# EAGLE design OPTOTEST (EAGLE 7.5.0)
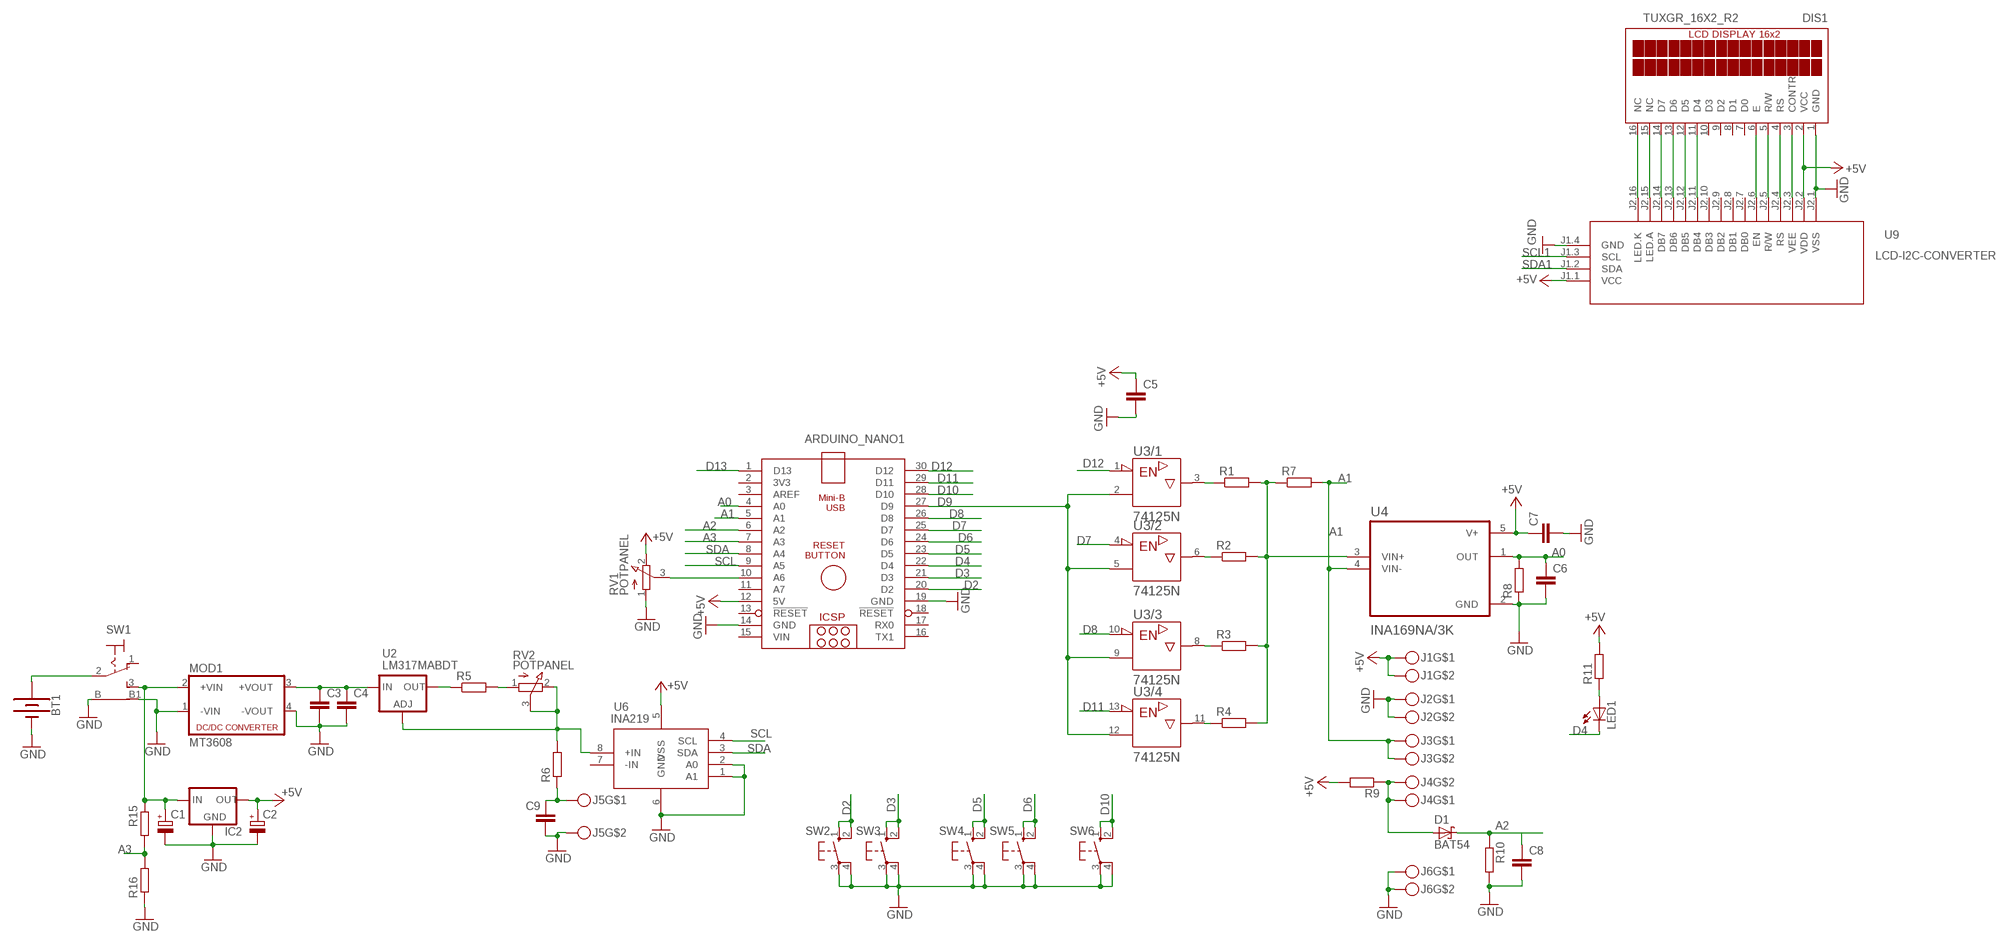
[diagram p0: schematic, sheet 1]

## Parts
ARDUINO_NANO1  ARDUINO_NANO  [ARDUINO_NANO]
BT1  BATTERY-9V  [BATTCON_9V]
C1  CPOL-EUSMCC  [SMC_C]
C2  CPOL-EUSMCC  [SMC_C]
C3  C-EUC1206  [C1206]
C4  C-EUC1206  [C1206]
C5  C-EUC1206  [C1206]
C6  C-EUC1206  [C1206]
C7  C-EUC1206  [C1206]
C8  C-EUC1206  [C1206]
C9  C-EUC1206  [C1206]
D1  BAT54  [SOT23]
DIS1  TUXGR_16X2_R2  [TUXGR_16X2_R2]
IC2  78XXL  [78XXL]
J1  MKDSN1,5-2-5,08  [MKDSN1,5-2-5,08]
J2  MKDSN1,5-2-5,08  [MKDSN1,5-2-5,08]
J3  MKDSN1,5-2-5,08  [MKDSN1,5-2-5,08]
J4  MKDSN1,5-2-5,08  [MKDSN1,5-2-5,08]
J5  MKDSN1,5-2-5,08  [MKDSN1,5-2-5,08]
J6  MKDSN1,5-2-5,08  [MKDSN1,5-2-5,08]
LED1  LED5MM  [LED5MM]
MOD1  MT3608  [MT3608]
R1  R-EU_R1206  [R1206]
R2  R-EU_R1206  [R1206]
R3  R-EU_R1206  [R1206]
R4  R-EU_R1206  [R1206]
R5  R-EU_R2512  [R2512]
R6  R-EU_R2512  [R2512]
R7  R-EU_R1206  [R1206]
R8  R-EU_R1206  [R1206]
R9  R-EU_R1206  [R1206]
R10  R-EU_R1206  [R1206]
R11  R-EU_R1206  [R1206]
R15  R-EU_R1206  [R1206]
R16  R-EU_R1206  [R1206]
RV1  POTPANEL  [POTPANELP231]
RV2  POTPANEL  [POTPANELP231]
SW1  9070-1W  [9070-1W]
SW2  40-XX  [B3F-40XX]
SW3  40-XX  [B3F-40XX]
SW4  40-XX  [B3F-40XX]
SW5  40-XX  [B3F-40XX]
SW6  40-XX  [B3F-40XX]
U2  LM317MABDT  [DPACK]
U3  74125N  [DIL14]
U4  INA169NA/3K  [SOT95P280X145-5N]
U6  INA219  [SO08]
U9  LCD-I2C-CONVERTER  [LCD-I2C-CONVERTER]

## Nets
+5V: ARDUINO_NANO1.12(5V) C2.+ C5.1 C7.1 DIS1.2(VCC) IC2.OUT J1.1 J1.2 R9.2 R11.2 RV1.2(E) U4.5(V+) U6.5(VSS) U9.J1.1(VCC) U9.J2.2(VDD)
A0: ARDUINO_NANO1.4(A0) C6.1 R8.2 U4.1(OUT)
A1: ARDUINO_NANO1.5(A1) J3.1 J3.2 R7.2 U4.4(VIN-)
A2: ARDUINO_NANO1.6(A2) C8.1 D1.3(C) R10.1
A3: ARDUINO_NANO1.7(A3) R15.1 R16.2
D2: ARDUINO_NANO1.20(D2) SW2.1(S) SW2.2(S1)
D3: ARDUINO_NANO1.21(D3) SW3.1(S) SW3.2(S1)
D4: ARDUINO_NANO1.22(D4) LED1.K(C)
D5: ARDUINO_NANO1.23(D5) SW4.1(S) SW4.2(S1)
D6: ARDUINO_NANO1.24(D6) SW5.1(S) SW5.2(S1)
D7: ARDUINO_NANO1.25(D7) U3.4(/2:!G)
D8: ARDUINO_NANO1.26(D8) U3.10(/3:!G)
D9: ARDUINO_NANO1.27(D9) U3.2(/1:A) U3.5(/2:A) U3.9(/3:A) U3.12(/4:A)
D10: ARDUINO_NANO1.28(D10) SW6.1(S) SW6.2(S1)
D11: ARDUINO_NANO1.29(D11) U3.13(/4:!G)
D12: ARDUINO_NANO1.30(D12) U3.1(/1:!G)
D13: ARDUINO_NANO1.1(D13)
GND: ARDUINO_NANO1.14(GND) ARDUINO_NANO1.19(GND) BT1.- C1.- C2.- C3.2 C4.2 C5.2 C6.2 C7.2 C8.2 C9.2 DIS1.1(GND) IC2.GND J2.1 J2.2 J5.2 J6.1 J6.2 MOD1.1(-VIN) MOD1.4(-VOUT) R8.1 R10.2 R16.1 RV1.1(A) SW1.B SW1.B1 SW2.3(P) SW2.4(P1) SW3.3(P) SW3.4(P1) SW4.3(P) SW4.4(P1) SW5.3(P) SW5.4(P1) SW6.3(P) SW6.4(P1) U4.2(GND) U6.1(A1) U6.2(A0) U6.6(GND) U9.J1.4(GND) U9.J2.1(VSS)
N$1: ARDUINO_NANO1.10(A6) RV1.3(S)
N$2: D1.1(A) J4.1 J4.2 R9.1
N$3: R1.1 U3.3(/1:Y)
N$4: R2.1 U3.6(/2:Y)
N$5: R3.1 U3.8(/3:Y)
N$6: R4.1 U3.11(/4:Y)
N$7: R1.2 R2.2 R3.2 R4.2 R7.1 U4.3(VIN+)
N$8: LED1.A R11.1
N$14: C3.1 C4.1 MOD1.3(+VOUT) U2.3(IN)
N$15: R5.1 U2.4(OUT)
N$16: R5.2 RV2.1(A)
N$17: R6.2 RV2.2(E) RV2.3(S) U2.1(ADJ) U6.8(+IN)
N$18: C1.+ IC2.IN MOD1.2(+VIN) R15.2 SW1.3(S)
N$19: C9.1 J5.1 R6.1
N$21: BT1.+ SW1.2(P)
N$31: DIS1.3(CONTR) U9.J2.3(VEE)
N$32: DIS1.4(RS) U9.J2.4(RS)
N$33: DIS1.5(R/W) U9.J2.5(R/W)
N$34: DIS1.6(E) U9.J2.6(EN)
N$35: DIS1.14(D7) U9.J2.14(DB7)
N$36: DIS1.13(D6) U9.J2.13(DB6)
N$37: DIS1.12(D5) U9.J2.12(DB5)
N$38: DIS1.11(D4) U9.J2.11(DB4)
N$39: DIS1.16(NC) U9.J2.16(LED.K)
N$40: DIS1.15(NC) U9.J2.15(LED.A)
SCL: ARDUINO_NANO1.9(A5) U6.4(SCL)
SCL1: U9.J1.3(SCL)
SDA: ARDUINO_NANO1.8(A4) U6.3(SDA)
SDA1: U9.J1.2(SDA)
Unconnected: ARDUINO_NANO1.2(3V3) ARDUINO_NANO1.3(AREF) ARDUINO_NANO1.11(A7) ARDUINO_NANO1.13(!RESET) ARDUINO_NANO1.16(TX1) ARDUINO_NANO1.17(RX0) ARDUINO_NANO1.18(!RESET) DIS1.7(D0) DIS1.8(D1) DIS1.9(D2) DIS1.10(D3) SW1.1(O) U6.7(-IN) U9.J2.7(DB0) U9.J2.8(DB1) U9.J2.9(DB2) U9.J2.10(DB3)

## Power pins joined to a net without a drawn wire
+UB: U3.14(/+UB:+UB)
-UB: U3.7(/-UB:-UB)
VIN: ARDUINO_NANO1.15(VIN)

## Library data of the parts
ARDUINO_NANO1 = ArduinoNanoV30:ARDUINO_NANO: Arduino Nano V3.0 Overview: The Arduino Nano is a small, complete, and breadboard-friendly board based on the ATmega328 (Arduino Nano 3.x) or ATmega168 (Arduino Nano 2.x). It has more or less the same functionality of the Arduino Duemilanove, but in a different package. It lacks only a DC power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
BT1 = SparkFun-Batteries:BATTERY: Battery - Single Cell; PROD_ID: BATT-10855
C1 C2 = rcl:CPOL-EU: POLARIZED CAPACITOR, European symbol
C3-C9 = rcl:C-EU: CAPACITOR, European symbol
D1 = diode:BAT54: Schottky Diodes
DIS1 = display-lcd:TUXGR_16X2_R2: Tuxgraphics LCD display 16x2 characters reflective, without background light Source: tuxgr_12x2_r2.pdf; OC_FARNELL: unknown; OC_NEWARK: unknown
IC2 = v-reg:78XXL: VOLTAGE REGULATOR
J1-J6 = con-phoenix-508:MKDSN1,5-2-5,08
LED1 = led:LED: LED
MOD1 = dc-dc-converter:MT3608: DC DC Up Converter
R1-R11 R15 R16 = rcl:R-EU_: RESISTOR, European symbol
RV1 RV2 = pot:POTPANEL
SW1 = switch:9070-1W: TOGGLE SWITCH Marquardt
SW2-SW6 = switch-omron:40-XX: OMRON SWITCH; MF: OMRON COMPONENTS USA; MPN: B3F-4000; OC_FARNELL: 176434; OC_NEWARK: 36K3105
U2 = v-reg:LM317?*: 500 mA Adjustable Output Positive Voltage Regulator Source: http://www.onsemi.co.jp .. LM317M-D.PDF
U3 = 74ttl-din:74*125: Quad bus BUFFER, 3-state
U4 = INA169NA_3K:INA169NA/3K: Check availability; AVAILABILITY: In Stock; CHECK_PRICES: https://www.snapeda.com/parts/INA169NA/3K/Texas+Instruments/view-part/?ref=eda; DESCRIPTION: 2.7 to 60V, 440kHz Variable gain current sense amplifier; MF: Texas Instruments; MP: INA169NA/3K; PACKAGE: SOT-23-5 Texas Instruments; PRICE: None; PURCHASE-URL: https://pricing.snapeda.com/search?q=INA169NA/3K&ref=eda; SNAPEDA_LINK: https://www.snapeda.com/parts/INA169NA/3K/Texas+Instruments/view-part/?ref=snap
U6 = burr-brown:INA219: Bidirectional Current/Power Monitor With I2C Interface
U9 = diy-modules:LCD-I2C-CONVERTER: I2C Bus to 4-Bit Parallel LCD Interface with LED backlight driver

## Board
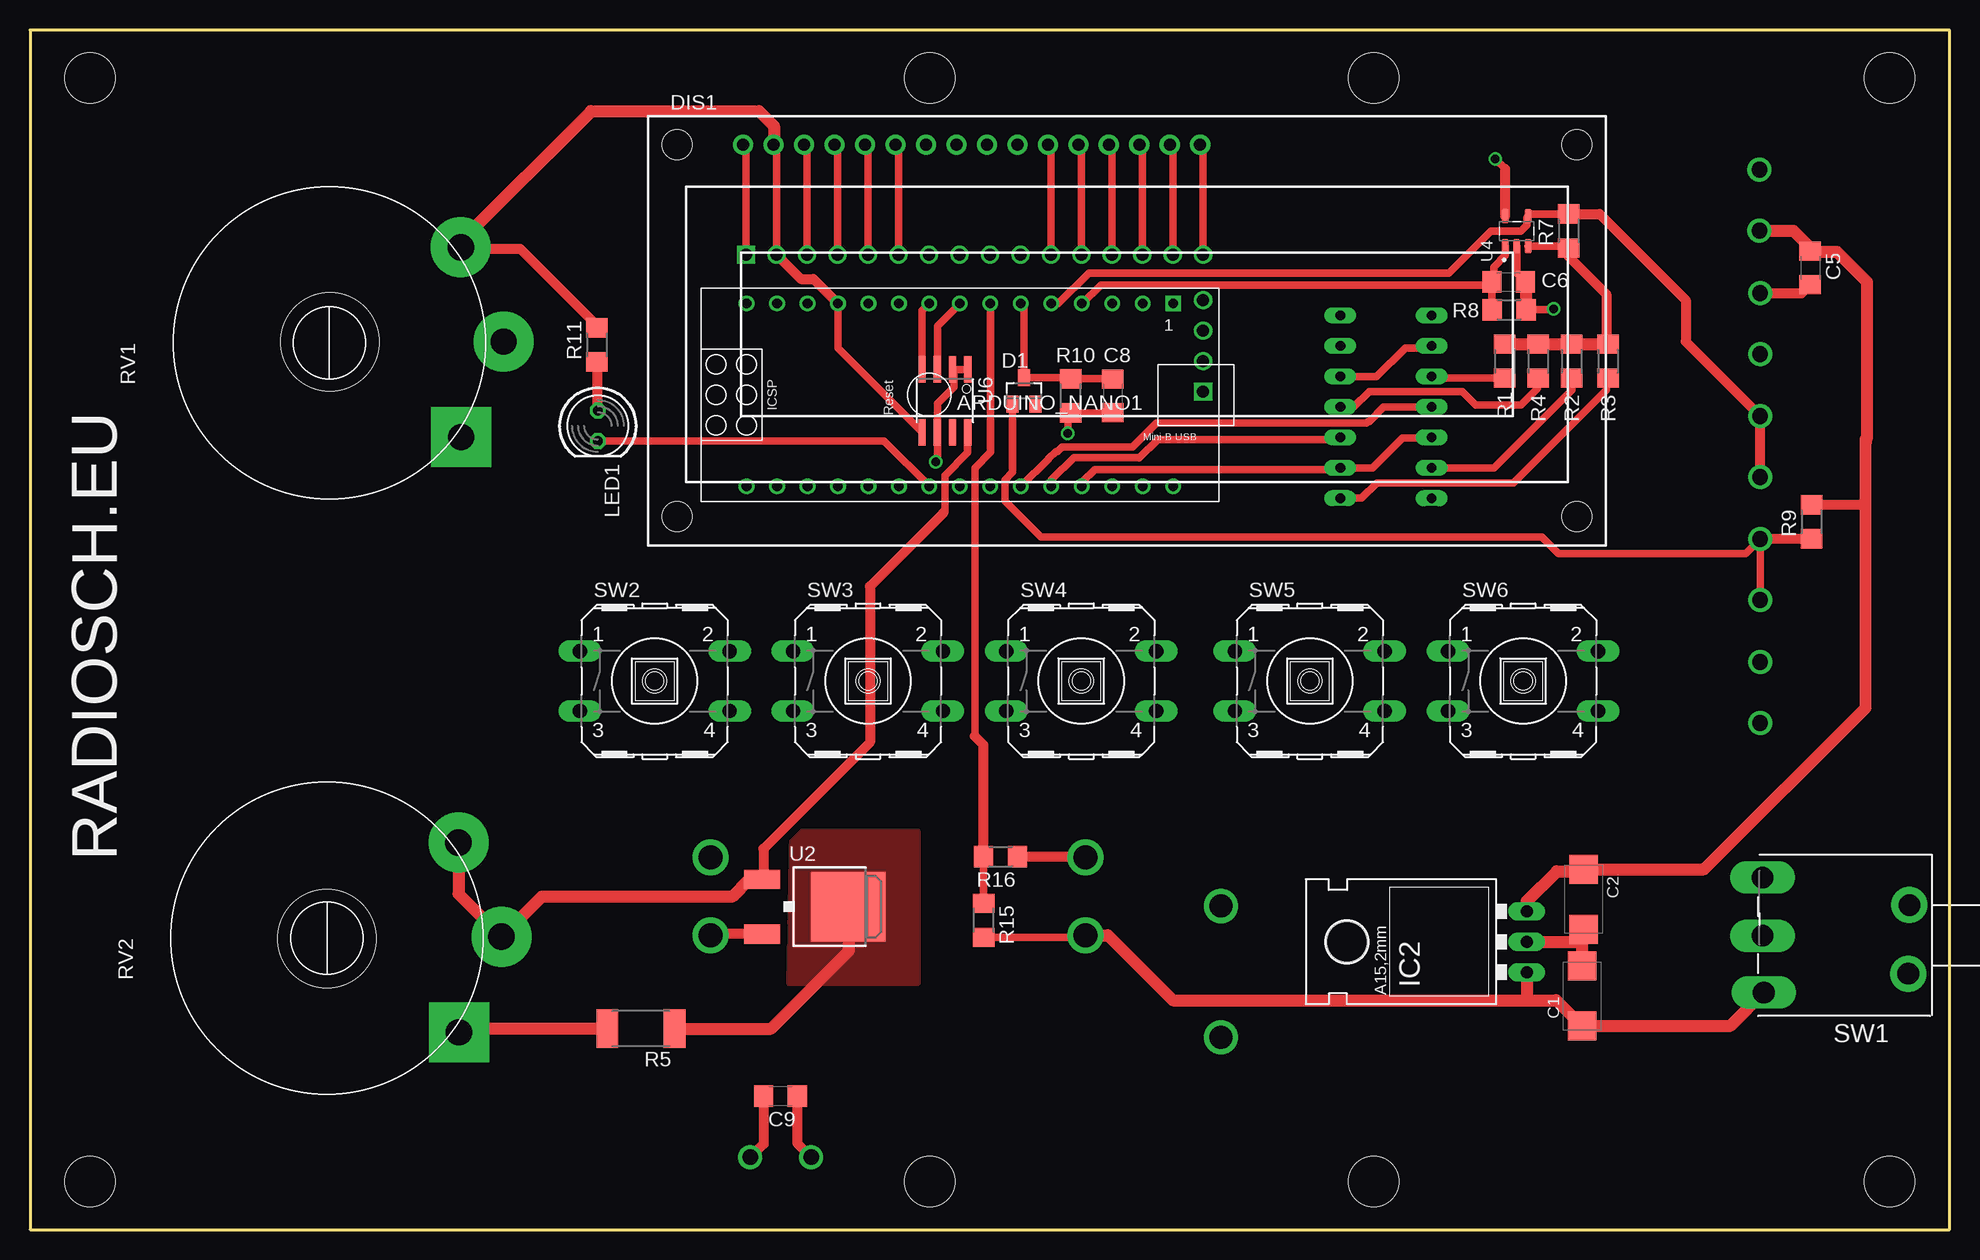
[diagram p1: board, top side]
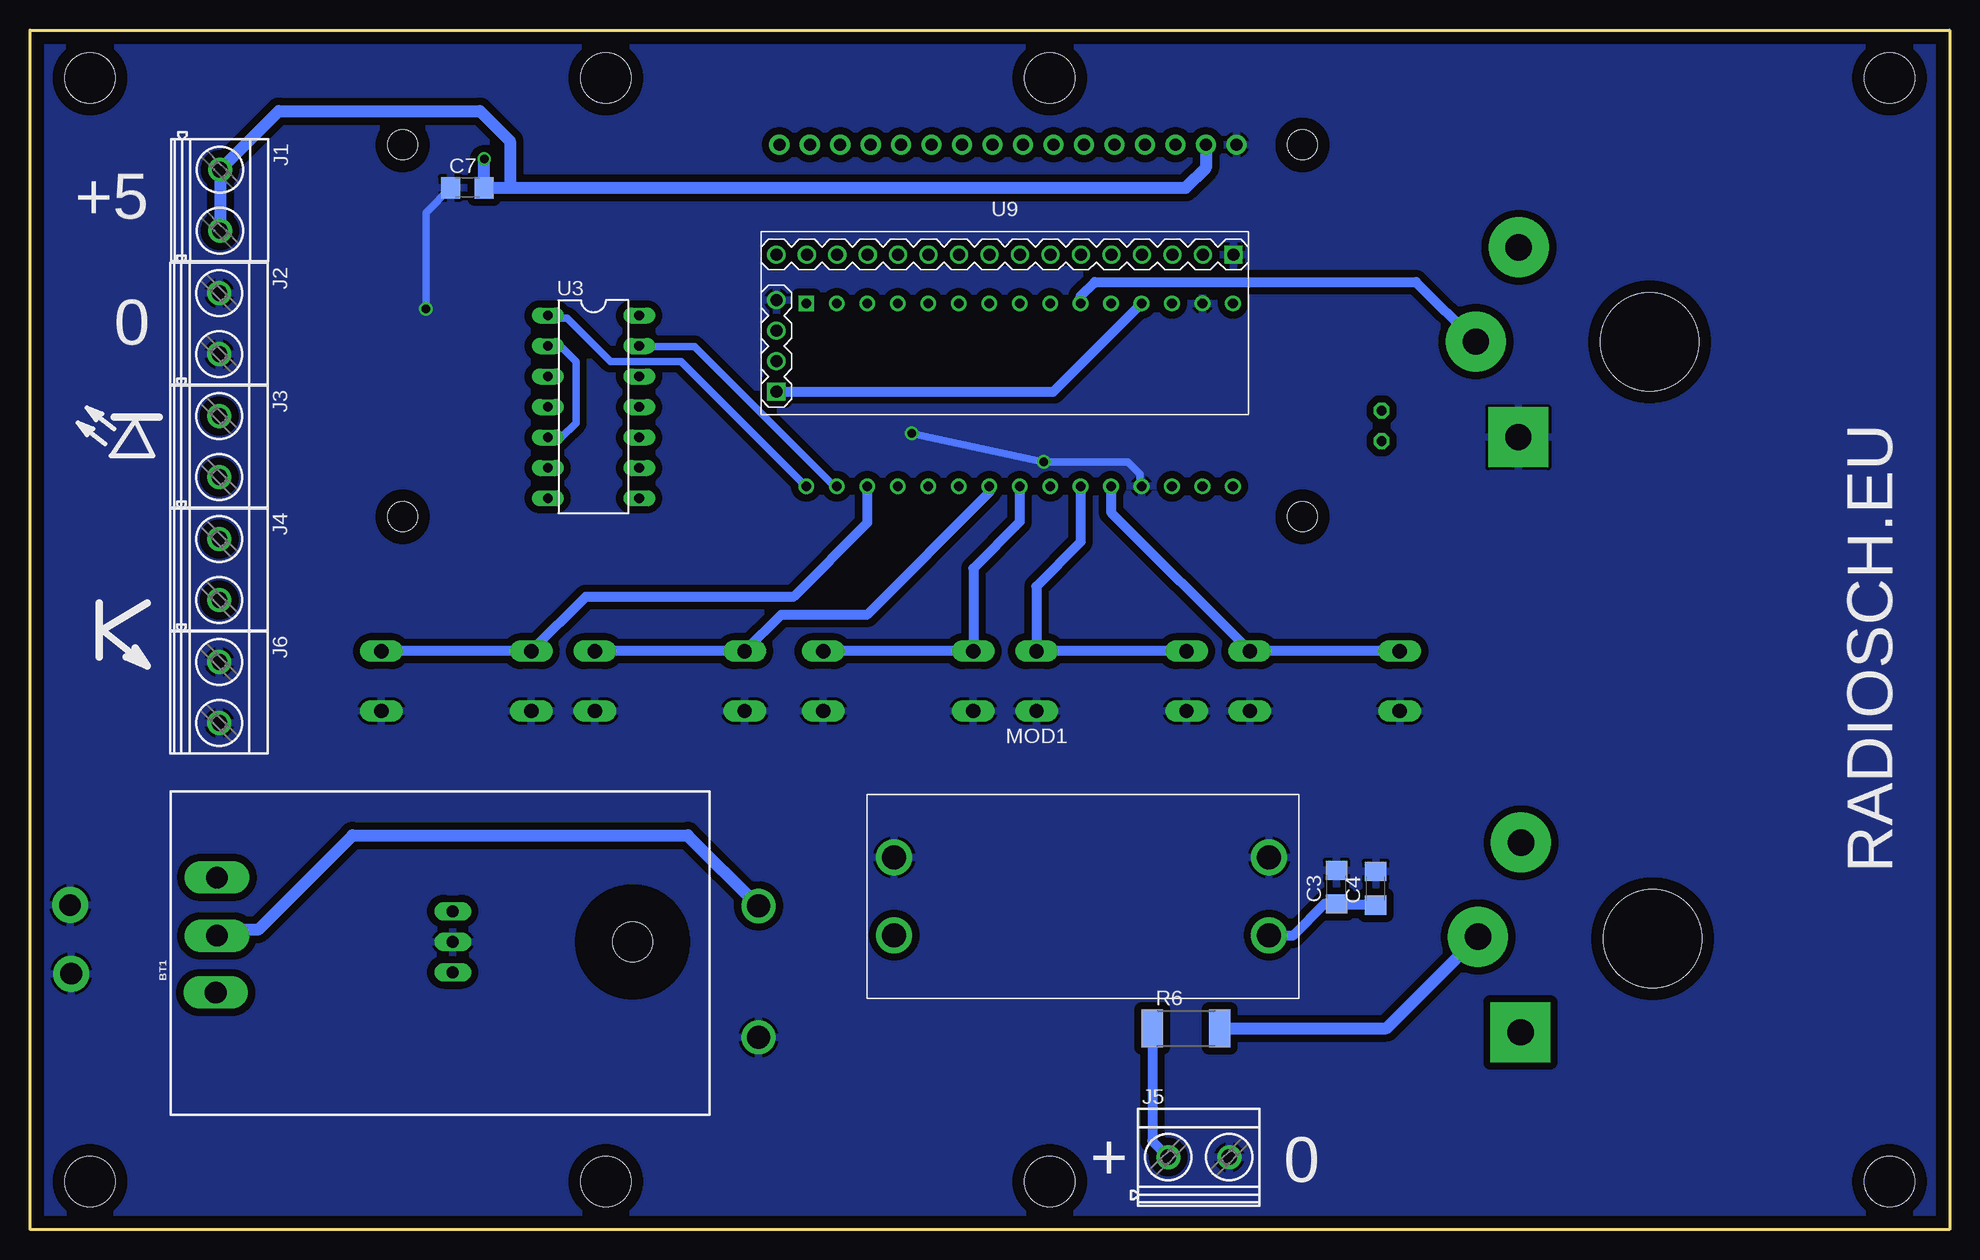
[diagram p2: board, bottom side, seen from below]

Size 160 x 100 mm. Coordinates in mm from the lower left corner, seen from the top.
Outline: 0,0 160,0 160,100 0,100 0,0
Copper layers (1*16): Top 0.035mm / dielectric 1.5mm / Bottom 0.035mm
Design rules "default": minimum track width 10mil, minimum drill 24mil, track to track 8mil, track to pad 8mil, pad to pad 8mil, via to via 8mil, smd to smd 8mil, copper to edge 40mil, drill to drill 8mil, minimum pad ring 10mil, minimum via ring 8mil, stop-mask expansion 4mil, vias tented up to drill 0mil, thermal gap 10mil
Holes 4.2 mm at 5,96 75,96 112,96 155,96 5,4 75,4 112,4 155,4
Holes 8.2 mm at 24.75,24.25 25,74

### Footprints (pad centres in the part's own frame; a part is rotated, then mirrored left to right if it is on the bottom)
ARDUINO_NANO = drill 0.8 square: 1 -20.32,-7.62 | drill 0.8: 2 -17.78,-7.62; 3 -15.24,-7.62; 4 -12.7,-7.62; 5 -10.16,-7.62; 6 -7.62,-7.62; 7 -5.08,-7.62; 8 -2.54,-7.62; 9 0,-7.62; 10 2.54,-7.62; 11 5.08,-7.62; 12 7.62,-7.62; 13 10.16,-7.62; 14 12.7,-7.62; 15 15.24,-7.62; 16 15.24,7.62; 17 12.7,7.62; 18 10.16,7.62; 19 7.62,7.62; 20 5.08,7.62; 21 2.54,7.62; 22 0,7.62; 23 -2.54,7.62; 24 -5.08,7.62; 25 -7.62,7.62; 26 -10.16,7.62; 27 -12.7,7.62; 28 -15.24,7.62; 29 -17.78,7.62; 30 -20.32,7.62
BATTCON_9V = drill 1.905: + -4,-1; - -4,-11.954
SMC_C = smd 2.4 x 2.4: + -2.5,0; - 2.5,0
C1206 = smd 1.6 x 1.8: 1 -1.4,0; 2 1.4,0
SOT23 = smd 1 x 1.4: 1 -0.95,-1.1; 2 0.95,-1.1; 3 0,1.1
TUXGR_16X2_R2 = drill 1 pad 1.676: 1 -32,15.5; 2 -29.46,15.5; 3 -26.92,15.5; 4 -24.38,15.5; 5 -21.84,15.5; 6 -19.3,15.5; 7 -16.76,15.5; 8 -14.22,15.5; 9 -11.68,15.5; 10 -9.14,15.5; 11 -6.6,15.5; 12 -4.06,15.5; 13 -1.52,15.5; 14 1.02,15.5; 15 3.56,15.5; 16 6.1,15.5 | hole 2.5: -37.5,-15.5; 37.5,-15.5; -37.5,15.5; 37.5,15.5
78XXL = drill 1.016 long: GND 0,-3.81; IN -2.54,-3.81; OUT 2.54,-3.81 | hole 3.302: 0,11.176
MKDSN1,5-2-5,08 = drill 1.3 pad 2: 1 -2.561,0.025; 2 2.519,0.025
LED5MM = drill 0.813 octagon: A -1.27,0; K 1.27,0
MT3608 = drill 2: 1 2.25,11.75; 2 2.25,5.25; 3 33.5,5.25; 4 33.5,11.75
R1206 = smd 1.6 x 1.803: 1 -1.422,0; 2 1.422,0
R2512 = smd 1.8 x 3.2: 1 -2.8,0; 2 2.8,0
POTPANELP231 = drill 2.2 pad 5 square: 1 -7.85,-11 | drill 2.2 pad 5: 2 7.97,-10.96; 3 0.11,-14.54
9070-1W = drill 1.813 long: 1 5.08,-4.835; 2 5.08,0 | drill 1.8 long: 3 4.98,4.735 | drill 1.8 pad 3: B -7.161,-2.544; B1 -7.061,3.167
B3F-40XX = drill 1.194 long: 1 -6.248,2.489; 2 6.248,2.489; 3 -6.248,-2.489; 4 6.248,-2.489
DPACK = smd 1.6 x 3: 1 -2.28,-4.8; 3 2.28,-4.8 | smd 5.8 x 6.2: 4 0,2.38
DIL14 = drill 0.813 long: 1 -7.62,-3.81; 2 -5.08,-3.81; 3 -2.54,-3.81; 4 0,-3.81; 5 2.54,-3.81; 6 5.08,-3.81; 7 7.62,-3.81; 8 7.62,3.81; 9 5.08,3.81; 10 2.54,3.81; 11 0,3.81; 12 -2.54,3.81; 13 -5.08,3.81; 14 -7.62,3.81
SOT95P280X145-5N = smd 1.21 x 0.59: 1 -1.255,0.95; 2 -1.255,0; 3 -1.255,-0.95; 4 1.255,-0.95; 5 1.255,0.95
SO08 = smd 0.61 x 2.21: 1 -1.905,-2.616; 2 -0.635,-2.616; 3 0.635,-2.616; 4 1.905,-2.616; 5 1.905,2.616; 6 0.635,2.616; 7 -0.635,2.616; 8 -1.905,2.616
LCD-I2C-CONVERTER = drill 1 square: J1.1 -19.05,-5.08; J2.1 19.05,6.35 | drill 1: J1.2 -19.05,-2.54; J1.3 -19.05,0; J1.4 -19.05,2.54; J2.2 16.51,6.35; J2.3 13.97,6.35; J2.4 11.43,6.35; J2.5 8.89,6.35; J2.6 6.35,6.35; J2.7 3.81,6.35; J2.8 1.27,6.35; J2.9 -1.27,6.35; J2.10 -3.81,6.35; J2.11 -6.35,6.35; J2.12 -8.89,6.35; J2.13 -11.43,6.35; J2.14 -13.97,6.35; J2.15 -16.51,6.35; J2.16 -19.05,6.35

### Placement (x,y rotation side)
ARDUINO_NANO1  74.97,69.58 180 top
BT1  95.27,27.97 0 bottom
C1  129.38,19.47 90 top
C2  129.5,27.53 270 top
C3  51.09,28.55 90 bottom
C4  47.83,28.45 90 bottom
C5  148.38,80.17 270 top
C6  123.25,79 0 top
C7  123.54,86.85 180 bottom
C8  90.25,69.5 270 top
C9  62.55,11.12 180 top
D1  82.85,69.92 0 top
DIS1  91.44,74.93 0 top
IC2  120.95,23.99 90 top
J1  144.18,85.79 270 bottom
J2  144.25,75.5 270 bottom
J3  144.25,65.25 270 bottom
J4  144.25,55 270 bottom
J5  62.56,6.01 0 bottom
J6  144.25,44.75 270 bottom
LED1  47.33,67 270 top
MOD1  90.21,19.28 0 bottom
R1  122.92,72.39 90 top
R2  128.5,72.39 90 top
R3  131.54,72.39 90 top
R4  125.71,72.39 90 top
R5  50.93,16.75 180 top
R6  63.65,16.77 0 bottom
R7  128.25,83.24 90 top
R8  123.29,76.68 180 top
R9  148.5,59 90 top
R10  86.75,69.5 270 top
R11  47.25,73.75 90 top
R15  79.49,25.77 270 top
R16  80.89,31.09 180 top
RV1  24.94,73.91 90 top
RV2  24.76,24.29 90 top
SW1  149.5,24.5 180 top
SW2  52.07,45.72 0 top
SW3  69.85,45.72 0 top
SW4  87.63,45.72 0 top
SW5  106.68,45.72 0 top
SW6  124.46,45.72 0 top
U2  65.82,26.91 270 top
U3  113.03,68.58 270 bottom
U4  123.92,83.24 90 top
U6  76.26,69.08 180 top
U9  78.74,74.93 0 bottom

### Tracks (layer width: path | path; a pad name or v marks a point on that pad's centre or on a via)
+5V  (via drill 0.7)
  Top 0.61: U9.J2.2 62.23,90.18 DIS1.2 | ARDUINO_NANO1.12 67.35,73.47 U6.5 | 122.97,88.42 v122.14,89.25
  Top 0.813: U9.J2.2 64.25,79.25 65.3,79.25 ARDUINO_NANO1.12 | 148.38,81.87 C5.1 148.45,81.5 | 144.18,83.25 J1.2 | 153.12,65.62 153.12,66 | R9.2 152.7,60.42 153,60.12 | R11.2 47.25,75.38 40.88,81.75 36.03,81.75 RV1.2 | U4.5 122.97,88.42
  Top 1.016: RV1.2 35.9,82.4 46.75,93.25 60.75,93.25 62,92 62,90.45 DIS1.2 | 148.38,81.87 147,83.25 144.18,83.25 | 148.45,81.5 150.62,81.5 153.12,79 153.12,66 153,65.88 153,60.12 153,43.5 139.53,30.03 130,30.03 | C2.+ 130,30.03 | IC2.OUT 124.76,27.39 127.25,29.88 128.75,29.88 129,29.62 129.59,29.62 130,30.03
  Bottom 0.813: 62,90.45 DIS1.2 | U9.J1.1 74.7,69.85 ARDUINO_NANO1.12
  Bottom 1.016: J1.2 J1.1 139.26,93.25 122.5,93.25 120,90.75 120,87.1 119.75,86.85 | 62,90.45 62,88.5 63.65,86.85 119.75,86.85 | 119.75,86.85 C7.1 v122.14,89.25
A0
  Top 0.61: ARDUINO_NANO1.4 87.7,77.2 89.25,78.75 121.6,78.75 C6.1 | R8.2 121.87,78.98 C6.1 | U4.1 122.97,81.22 122,80.25 122,79.15 C6.1
A1
  Top 0.61: ARDUINO_NANO1.5 85.7,77.2 88.25,79.75 118.25,79.75 121.75,83.25 124.25,83.25 124.75,83.75 124.75,84.38 U4.4 125.04,84.66 R7.2
  Top 0.813: J3.2 J3.1 138,74.04 138,77.5 130.84,84.66 R7.2
A2
  Top 0.61: ARDUINO_NANO1.6 82.85,76.94 D1.3 86.65,71.02 R10.1 90.23,70.92 C8.1
A3
  Top 0.61: 78.75,41.12 78.75,63.5 80.05,64.8 ARDUINO_NANO1.7 | R15.1 79.49,31.07 R16.2
  Top 0.813: R16.2 79.47,40.4 78.75,41.12
D2
  Bottom 0.813: ARDUINO_NANO1.20 69.89,59.78 SW2.2 SW2.1
D3
  Bottom 0.813: ARDUINO_NANO1.21 72.43,57.32 76.12,53.62 76.12,48.24 SW3.2 SW3.1
D4
  Top 0.61: LED1.K 71.2,65.73 ARDUINO_NANO1.22
D5
  Bottom 0.813: ARDUINO_NANO1.23 77.51,58.99 81.38,55.12 SW4.1 SW4.2
D6
  Bottom 0.813: ARDUINO_NANO1.24 80.05,61.45 90.25,51.25 97.39,51.25 SW5.1 SW5.2
D7
  Top 0.61: U3.4 112.83,68.58 111.62,67.38 111.5,67.38 111.38,67.25 93.88,67.25 91.88,65.25 86,65.25 85.62,64.88 85.5,64.88 84.88,64.25 ARDUINO_NANO1.25
D8
  Top 0.61: ARDUINO_NANO1.26 85.13,62.51 87,64.38 92.38,64.38 92.44,64.31 94,65.88 109.06,65.88 U3.10
D9
  Top 0.61: U3.12 112.25,71.12 114.62,73.5 116.68,73.5 U3.2 | 109.09,63.62 U3.9 | ARDUINO_NANO1.27 87.67,62.3 88.75,63.38 109.09,63.38 U3.9 | U3.9 111.88,63.5 114.38,66 116.8,66 U3.5
  Bottom 0.61: U3.5 115.71,66.04 114.5,67.25 114.5,72.38 115.62,73.5 116.68,73.5 U3.2
D10
  Bottom 0.813: ARDUINO_NANO1.28 90.21,58.91 96.38,52.75 113.67,52.75 SW6.1 SW6.2
D11
  Bottom 0.61: ARDUINO_NANO1.29 92.96,61.96 104.62,73.62 109.19,73.62 U3.13
D12
  Bottom 0.61: ARDUINO_NANO1.30 95.33,61.96 105.75,72.38 111.62,72.38 115.25,76 116.64,76 U3.1
GND  (via drill 0.7)
  Top 0.61: U9.J2.1 59.69,90.18 DIS1.1 | U6.1 U6.2 77,71.59 77,70.25 75.62,68.88 U6.6 75.62,64.12 v75.5,64 | v86.5,66.38 86.5,67.83 R10.2 90.23,68.08 C8.2 | U4.2 123.92,79.73 C6.2 | R8.1 126.93,76.68 v127,76.75
  Top 0.813: J2.1 147.67,78.06 C5.2 | R16.1 87.9,31.09 MOD1.1 | C9.2 61.15,7.14 J5.2
  Top 1.016: C1.- 129.38,23.75 | 129.38,23.75 129.38,24.91 C2.- | IC2.GND 129.14,23.99 129.38,23.75 | R8.1 124.71,78.94 C6.2
  Bottom 0.61: ARDUINO_NANO1.19 67.5,62.11 67.5,63 68.5,64 v75.5,64 v86.5,66.38 | v127,76.75 127,84.79 C7.2
  pour Bottom (isolate 0.61): 0,99 159,99 159,0.5 0,0.5
N$1
  Bottom 0.813: ARDUINO_NANO1.10 72.43,77.82 71.25,79 44.46,79 RV1.3
N$2
  Top 0.61: D1.1 81.9,63.15 81.25,62.5 81.25,60.75 84.25,57.75 126,57.75 127.38,56.38 143.04,56.38 J4.1 J4.2
  Top 0.813: R9.1 144.24,57.58 J4.1
N$3
  Top 0.61: R1.1 116.99,70.97 U3.3
N$4
  Top 0.61: R2.1 128.5,70 122,63.5 U3.6
N$5
  Top 0.61: U3.8 110.96,60.96 112.25,62.25 123.62,62.25 131.38,70 131.38,70.8 R3.1
N$6
  Top 0.61: U3.11 110.33,68.58 111.62,69.88 119.38,69.88 120.5,68.75 124.25,68.75 125.62,70.12 125.62,70.88 R4.1
N$7
  Top 0.61: U4.3 128.08,81.98 R7.1
  Top 0.813: R7.1 128.25,81.12 131.38,78 131.38,73.98 R3.2
  Top 1.016: R1.2 R4.2 R2.2 R3.2
N$8
  Top 0.813: R11.1 47.25,68.35 LED1.A
N$14
  Top 0.813: U2.3 56.81,24.63 MOD1.3
  Bottom 0.813: C4.1 50.99,27.05 C3.1 52.1,27.15 54.75,24.5 56.68,24.5 MOD1.3
N$15
  Top 1.016: R5.1 61.75,16.75 68.25,23.25 68.25,26.86 U2.4
  pour Top (isolate 0.61, no thermals): 64,33.25 74,33.25 74,20.5 63.25,20.5 63.5,33.25
N$16
  Top 1.016: R5.2 36.07,16.75 RV2.1
N$17
  Top 0.61: U6.8 78.17,64.79 76.25,62.88 76.25,59.88 76.12,59.75
  Top 0.813: 76.12,59.75 70,53.62 70,40.62 61.12,31.75 61.12,29.3 U2.1
  Top 1.016: U2.1 59.94,29.19 58.5,27.75 42.65,27.75 RV2.3 35.72,27.98 RV2.2
  Bottom 1.016: R6.2 46.92,16.77 RV2.3
N$18
  Top 0.61: R15.2 87.78,24.35 MOD1.2
  Top 1.016: MOD1.2 89.84,24.53 95.25,19.12 125,19.12 | 125,19.12 127.22,19.12 129.35,17 | 129.35,17 C1.+ | IC2.IN 124.76,19.36 125,19.12 | 129.35,17 141.75,17 SW1.3
N$19
  Top 0.813: C9.1 63.95,7.21 J5.1
  Bottom 0.813: R6.1 66.45,7.36 J5.1
N$21
  Bottom 1.016: BT1.+ 105.17,32.88 133.12,32.88 141,25 143.92,25 SW1.2
N$31
  Top 0.61: U9.J2.3 64.77,90.18 DIS1.3
N$32
  Top 0.61: U9.J2.4 67.31,90.18 DIS1.4
N$33
  Top 0.61: U9.J2.5 69.85,90.18 DIS1.5
N$34
  Top 0.61: U9.J2.6 72.39,90.18 DIS1.6
N$35
  Top 0.61: U9.J2.14 92.71,90.18 DIS1.14
N$36
  Top 0.61: U9.J2.13 90.17,90.18 DIS1.13
N$37
  Top 0.61: U9.J2.12 87.63,90.18 DIS1.12
N$38
  Top 0.61: U9.J2.11 85.09,90.18 DIS1.11
N$39
  Top 0.61: U9.J2.16 97.79,90.18 DIS1.16
N$40
  Top 0.61: U9.J2.15 95.25,90.18 DIS1.15
SCL
  Top 0.61: U6.4 74.36,76.58 ARDUINO_NANO1.9
SDA
  Top 0.61: U6.3 75.62,75.31 ARDUINO_NANO1.8

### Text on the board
tPlace: RADIOSCH.EU
bPlace: +5 | 0 | RADIOSCH.EU | 0 | +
